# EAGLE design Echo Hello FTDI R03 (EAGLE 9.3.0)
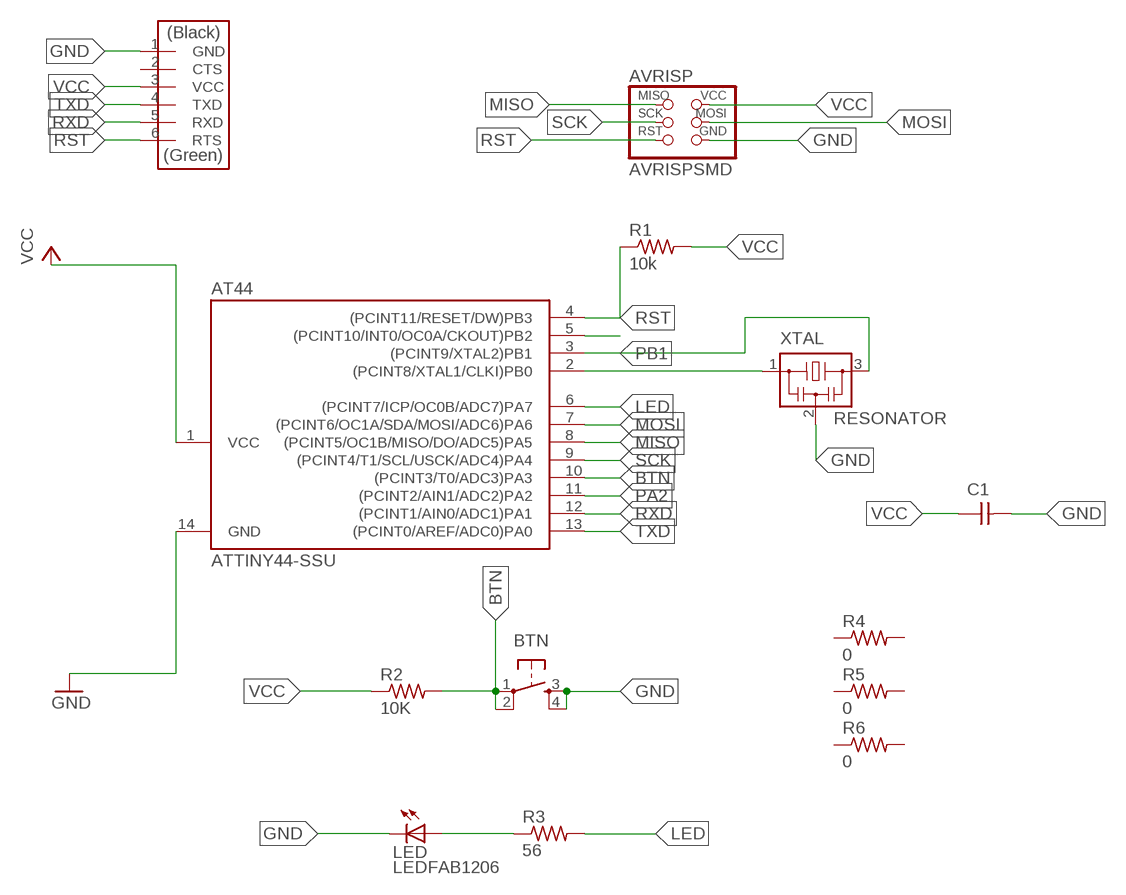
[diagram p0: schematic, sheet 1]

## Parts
AT44  ATTINY44-SSU  [SOIC14]
AVRISP  AVRISPSMD  [2X03SMD]
BTN  6MM_SWITCH6MM_SWITCH  [6MM_SWITCH]
C1  CAP-UNPOLARIZEDFAB  [C1206FAB]
FTDI  FTDI-SMD-HEADER  [1X06SMD]
LED  LEDFAB1206  [LED1206FAB]
R1  10k  RES-US1206FAB  [R1206FAB]
R2  10K  RES-US1206FAB  [R1206FAB]
R3  56  RES-US1206FAB  [R1206FAB]
R4  0  RES-US1206FAB  [R1206FAB]
R5  0  RES-US1206FAB  [R1206FAB]
R6  0  RES-US1206FAB  [R1206FAB]
XTAL  RESONATOR  [EFOBM]

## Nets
BTN: AT44.10((PCINT3/T0/ADC3)PA3) BTN.1(P) BTN.2(P1) R2.2
GND: AT44.14(GND) AVRISP.6(GND) BTN.3(S) BTN.4(S1) C1.2 FTDI.1(GND) LED.2(C) XTAL.2
LED: AT44.6((PCINT7/ICP/OC0B/ADC7)PA7) R3.2
MISO: AT44.8((PCINT5/OC1B/MISO/DO/ADC5)PA5) AVRISP.1(MISO)
MOSI: AT44.7((PCINT6/OC1A/SDA/MOSI/ADC6)PA6) AVRISP.4(MOSI)
N$1: AT44.2((PCINT8/XTAL1/CLKI)PB0) XTAL.1
N$6: AT44.5((PCINT10/INT0/OC0A/CKOUT)PB2)
N$11: LED.1(A) R3.1
PA2: AT44.11((PCINT2/AIN1/ADC2)PA2)
PB1: AT44.3((PCINT9/XTAL2)PB1) XTAL.3
RST: AT44.4((PCINT11/RESET/DW)PB3) AVRISP.5(RST) FTDI.6(RTS) R1.1
RXD: AT44.12((PCINT1/AIN0/ADC1)PA1) FTDI.5(RXD)
SCK: AT44.9((PCINT4/T1/SCL/USCK/ADC4)PA4) AVRISP.3(SCK)
TXD: AT44.13((PCINT0/AREF/ADC0)PA0) FTDI.4(TXD)
VCC: AT44.1(VCC) AVRISP.2(VCC) C1.1 FTDI.3(VCC) R1.2 R2.1
Unconnected: FTDI.2(CTS) R4.1 R4.2 R5.1 R5.2 R6.1 R6.2

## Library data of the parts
AT44 = fab:ATTINY44
AVRISP = fab:AVRISP
BTN = fab:6MM_SWITCH: OMRON SWITCH
C1 = fab:CAP-UNPOLARIZED
FTDI = fab:FTDI-SMD-HEADER
LED = fab:LED: LED
R1-R6 = fab:RES-US: Resistor (US Symbol)
XTAL = fab:RESONATOR

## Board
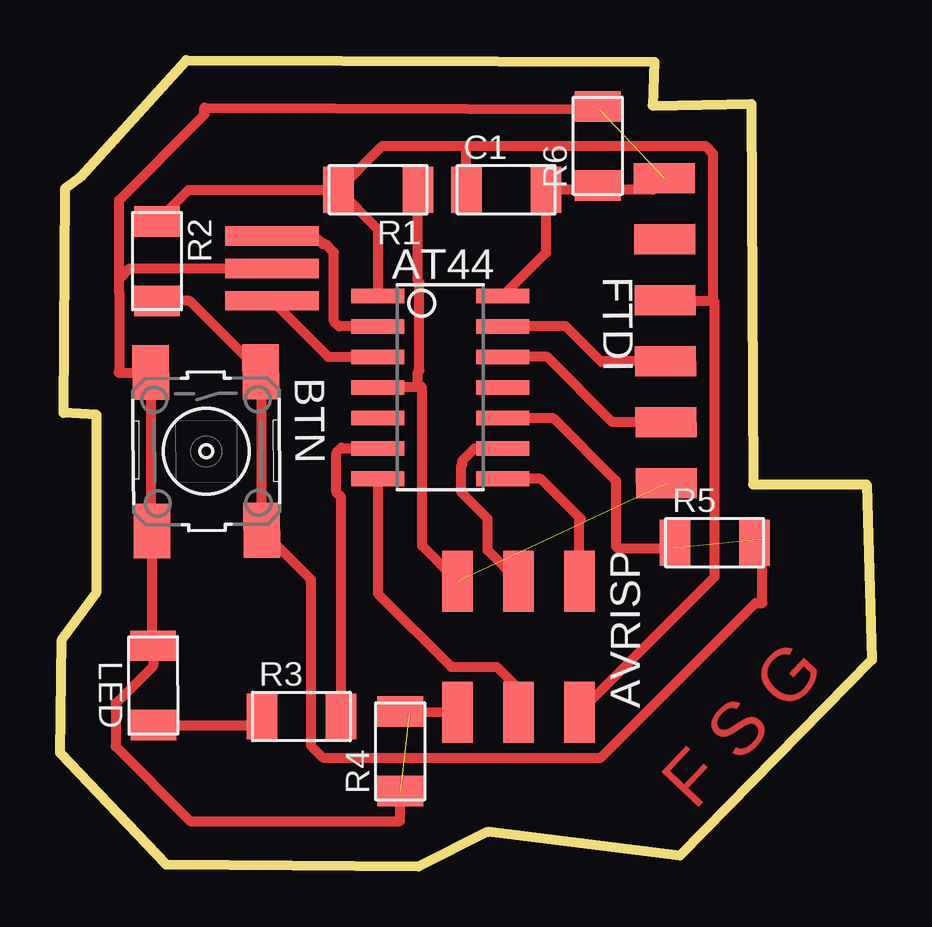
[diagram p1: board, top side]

Size 33.83 x 33.6 mm. Coordinates in mm from the lower left corner, seen from the top.
Outline: 0.84,28.73 5.26,33.6 24.76,33.53 24.69,31.7 28.8,31.78 28.88,15.93 33.6,15.93 33.83,8.61 25.83,0.46 17.83,1.45 14.94,0 4.42,0.08 0,4.72 0.08,9.45 1.52,11.43 1.52,18.82 0.15,18.9 0.23,28.27 0.84,28.73
Copper layers (1*16): Top 0.035mm / dielectric 1.5mm / Bottom 0.035mm
Design rules "fabmodule": minimum track width 10mil, minimum drill 0.4mm, track to track 0.42mm, track to pad 0.42mm, pad to pad 0.42mm, via to via 0.42mm, smd to smd 0.42mm, copper to edge 40mil, drill to drill 0.8mm, minimum pad ring 10mil, minimum via ring 8mil, stop-mask expansion 4mil, vias tented up to drill 0mil, thermal gap 10mil

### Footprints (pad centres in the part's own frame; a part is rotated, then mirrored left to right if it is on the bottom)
SOIC14 = smd 0.61 x 2.21: 1 -3.81,-2.603; 2 -2.54,-2.603; 3 -1.27,-2.603; 4 0,-2.603; 5 1.27,-2.603; 6 2.54,-2.603; 7 3.81,-2.603; 8 3.81,2.603; 9 2.54,2.603; 10 1.27,2.603; 11 0,2.603; 12 -1.27,2.603; 13 -2.54,2.603; 14 -3.81,2.603
2X03SMD = smd 2.54 x 1.27: 1 -2.54,2.54; 2 2.92,2.54; 3 -2.54,0; 4 2.92,0; 5 -2.54,-2.54; 6 2.92,-2.54
6MM_SWITCH = smd 2.286 x 1.524: 1 -3.302,2.286; 2 3.302,2.286; 3 -3.302,-2.286; 4 3.302,-2.286
C1206FAB = smd 1.27 x 1.905: 1 -1.651,0; 2 1.651,0
1X06SMD = smd 2.54 x 1.27: 1 0,6.35; 2 0,3.81; 3 0,1.27; 4 0,-1.27; 5 0,-3.81; 6 0,-6.35
LED1206FAB = smd 1.27 x 1.905: 1 -1.651,0; 2 1.651,0
R1206FAB = smd 1.27 x 1.905: 1 -1.651,0; 2 1.651,0
EFOBM = smd 0.8 x 3.9: 1 -1.35,0; 2 0,0; 3 1.35,0

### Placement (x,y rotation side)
AT44  15.85,19.96 270 top
AVRISP  19.1,9.35 270 top
BTN  6.1,17.3 270.4 top
C1  18.59,28.19 0 top
FTDI  25.22,22.33 0.4 top
LED  3.89,7.54 90.3 top
R1  13.26,28.19 180 top
R2  4.04,25.22 270 top
R3  10.06,6.25 0 top
R4  14.17,4.8 90 top
R5  27.28,13.49 0 top
R6  22.4,30.02 90 top
XTAL  8.84,24.92 270 top

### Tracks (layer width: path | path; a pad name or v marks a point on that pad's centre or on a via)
BTN  (1 unrouted)
  Top 0.406: R2.2 5.4,23.57 BTN.1 8.4,20.57 BTN.2 10.45,11.96 10.45,5.04 10.95,4.53 22.53,4.53 28.97,10.97 29.26,10.97 29.26,13.64 29.34,13.72 | AT44.10 20.55,18.69 23.16,16.08 23.16,13.33 23.24,13.26 25.6,13.26
GND  (2 unrouted)
  Top 0.406: FTDI.1 24.7,28.19 C1.2 20.24,25.56 AT44.14 | 2.46,24.46 2.92,24.92 XTAL.2 | AVRISP.6 14.55,6.4 | 14.17,3.12 14.17,1.89 5.42,1.89 2.31,5 2.31,6.78 3.88,8.34 LED.2 3.83,9.24 BTN.4 3.79,14.03 BTN.3 3.78,20.57 2.44,20.57 2.46,20.6 2.46,23.93 2.46,24.46 | 2.46,24.46 2.46,27.77 6.02,31.32 6.02,31.62 22.48,31.55
LED
  Top 0.406: R3.2 11.71,15.4 11.52,15.59 11.52,17.23 11.73,17.45 11.76,17.42 AT44.6
MISO
  Top 0.406: AVRISP.1 21.64,14.4 21.72,14.48 20.04,16.15 AT44.8
MOSI
  Top 0.406: AT44.7 13.25,11.37 16.29,8.32 18.2,8.32 19.35,7.16 19.1,6.91 AVRISP.4
N$1
  Top 0.406: AT44.2 11.63,22.5 11.41,22.72 11.41,25.58 11.05,25.94 10.94,25.94 10.59,26.29 10.57,26.27 XTAL.1
N$11
  Top 0.406: LED.1 8.05,5.89 R3.1
PB1
  Top 0.406: XTAL.3 11.17,21.23 AT44.3
RST  (1 unrouted)
  Top 0.406: AVRISP.5 15.09,13.36 15.09,19.96 | 15.09,19.96 AT44.4 | 15.09,19.96 14.91,20.14 14.91,20.61 14.97,20.67 14.97,24.34 14.91,24.4 R1.1
RXD
  Top 0.406: FTDI.5 23.01,18.52 20.29,21.23 AT44.12
SCK
  Top 0.406: AVRISP.3 17.82,13.17 17.82,14.5 16.72,15.59 16.72,16.72 16.76,16.76 16.76,16.92 17.27,17.42 AT44.9
TXD
  Top 0.406: FTDI.4 22.66,21.06 22.63,21.03 22.56,21.03 21.08,22.5 AT44.13
VCC
  Top 0.406: R2.1 5.36,28.19 R1.2 | R1.2 13.25,26.56 AT44.1 | R1.2 13.44,30.02 16.92,30.02 | 16.92,30.02 16.92,28.22 C1.1 | 16.92,30.02 26.9,30.02 27.2,29.72 27.2,23.62 27.28,23.55 | 27.28,23.55 25.26,23.55 FTDI.3 | AVRISP.2 27.28,12.07 27.28,23.55

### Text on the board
Top: F S G
201bmp: /Users/FelipeSG/Desktop/flash.BMP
